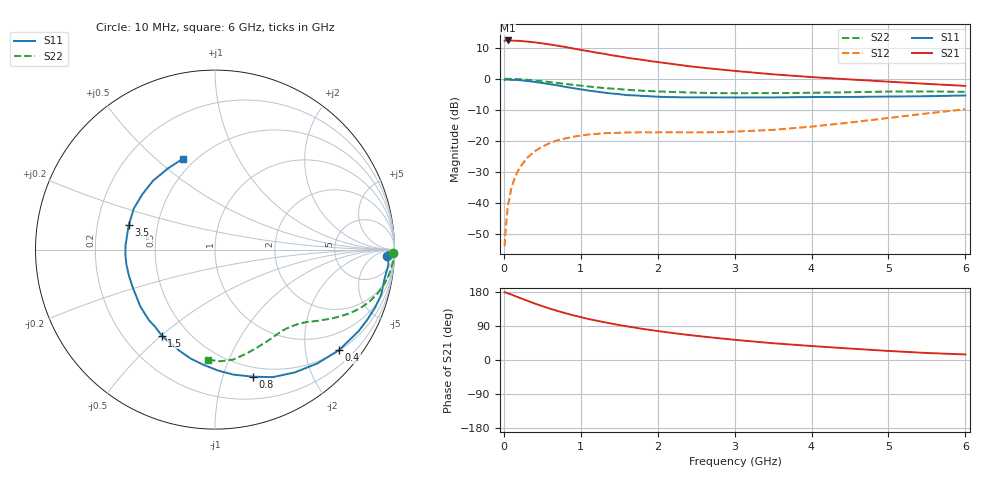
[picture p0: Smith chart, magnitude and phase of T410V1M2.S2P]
! Infineon Technologies  Discrete & RF Semiconductors
! BFR182T
! Si NPN RF Bipolar Junction Transistor in SC75
! VCE = 10 V  IC = 1.2 mA
! Common Emitter S-Parameters:  October  1999
# GHz  S  MA  R  50
!  f  S11  S21  S12  S22
! GHz  MAG  ANG  MAG  ANG  MAG  ANG  MAG  ANG
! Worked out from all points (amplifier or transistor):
!   36 points, 10 MHz to 6 GHz, reference 50 ohm
!   highest |S21| = 12.3 dB at 50 MHz (marker M1)
!   |S21| within 3 dB of that: start of sweep to 990.3 MHz
!   unconditionally stable (mu >= 1): 2.368 GHz to 4.605 GHz
!   at 250 MHz: K = 0.10, MSG = 19.6 dB, |S12| = -27.2 dB
!   at 1.4 GHz: K = 0.61, MSG = 12.5 dB, |S12| = -17.5 dB
!   at 6 GHz: K = 0.83, MSG = 3.8 dB, |S12| = -9.8 dB
!   S11 on the Smith chart (normalised r, x): 10 MHz: 27, -23; 400 MHz: 0.51, -2.74; 800 MHz: 0.40, -1.26; 1.5 GHz: 0.36, -0.50; 3.5 GHz: 0.34, +0.12; 6 GHz: 0.43, +0.61
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0.01  0.9582 -2.1  4.118 178.5  0.002 77.3  0.9904 -1.2
0.02  0.9628 -0.7  4.091 178.8  0.0032 94.6  0.9999 -0.9
0.05  0.9696 -5.0  4.139 176.1  0.0085 91.0  0.995 -2.0
0.1  0.9585 -9.6  4.104 172.6  0.0177 87.0  0.9937 -4.1
0.15  0.9595 -15.2  4.104 168.4  0.0269 81.2  0.9872 -6.0
0.25  0.9345 -24.6  4.03 160.7  0.0437 75.4  0.9717 -9.8
0.4  0.8897 -39.0  3.862 149.1  0.0675 67.6  0.938 -15.2
0.5  0.853 -48.0  3.717 142.2  0.0805 62.5  0.9115 -18.2
0.6  0.8159 -57.0  3.56 135.4  0.092 58.4  0.8821 -21.1
0.7  0.7803 -65.6  3.403 129.3  0.1023 54.6  0.853 -23.5
0.8  0.7394 -73.3  3.249 123.5  0.109 50.7  0.8239 -25.7
0.9  0.7045 -81.5  3.076 118.1  0.1158 47.7  0.7967 -27.6
1.1  0.6443 -95.9  2.787 108.2  0.1263 42.5  0.7499 -30.9
1.3  0.5975 -109.3  2.527 100.0  0.1323 38.8  0.7095 -33.7
1.5  0.5638 -121.7  2.293 92.3  0.1346 36.3  0.6796 -36.0
1.8  0.5279 -138.6  2.016 82.2  0.137 34.0  0.6401 -39.4
2.2  0.5041 -156.0  1.722 71.0  0.1371 34.0  0.6115 -43.6
2.8  0.5001 -176.9  1.415 57.4  0.1377 38.3  0.5865 -50.9
3.5  0.4997 164.2  1.178 44.2  0.1499 47.1  0.587 -59.6
4.5  0.5089 142.7  0.974 30.2  0.1969 56.9  0.6059 -73.4
5.5  0.5226 120.2  0.826 18.5  0.2758 58.8  0.6227 -87.2
6  0.5368 109.6  0.767 14.6  0.3223 56.7  0.6153 -93.7
